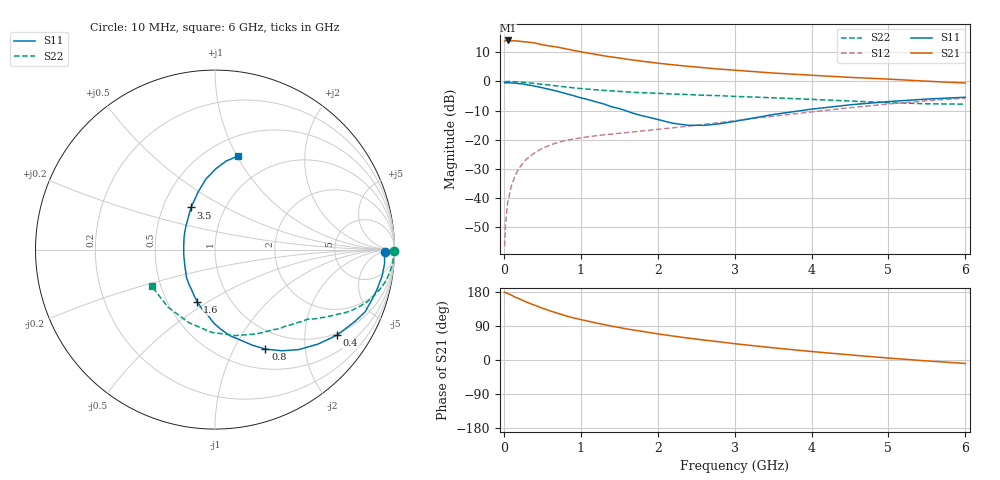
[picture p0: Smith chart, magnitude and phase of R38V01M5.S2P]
! SIEMENS Small Signal Semiconductors
! BFR181
! Si NPN RF Bipolar Junction Transistor in SOT23
! VCE = 8 V  IC = 1.5 mA
! Common Emitter S-Parameters:  May  1996
# GHz  S  MA  R  50
!  f  S11  S21  S12  S22
! GHz  MAG  ANG  MAG  ANG  MAG  ANG  MAG  ANG
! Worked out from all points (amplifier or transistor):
!   36 points, 10 MHz to 6 GHz, reference 50 ohm
!   highest |S21| = 14.0 dB at 50 MHz (marker M1)
!   |S21| within 3 dB of that: start of sweep to 830.6 MHz
!   unconditionally stable (mu >= 1): 1.833 GHz to 3.565 GHz
!   at 250 MHz: K = 0.19, MSG = 20.8 dB, |S12| = -27.9 dB
!   at 1.4 GHz: K = 0.86, MSG = 13.2 dB, |S12| = -18.1 dB
!   at 6 GHz: K = 0.86, MSG = 2.6 dB, |S12| = -5.7 dB
!   S11 on the Smith chart (normalised r, x): 10 MHz: 34, -10; 400 MHz: 0.94, -2.90; 800 MHz: 0.74, -1.35; 1.6 GHz: 0.70, -0.45; 3.5 GHz: 0.69, +0.35; 6 GHz: 0.69, +1.01
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0.01  0.9475 -0.9  4.937 179.0  0.0015 89.8  0.9981 -0.5
0.02  0.9451 -1.8  4.979 177.8  0.0033 91.1  0.9883 -0.9
0.05  0.9481 -4.7  5.032 175.4  0.0084 87.4  0.9956 -2.2
0.1  0.9423 -9.1  4.944 171.1  0.0164 83.0  0.9931 -4.3
0.15  0.9292 -14.0  4.969 165.5  0.0249 81.0  0.9845 -6.6
0.3  0.8775 -27.0  4.743 152.4  0.0472 73.7  0.9524 -12.6
0.4  0.8307 -35.0  4.563 144.8  0.0597 68.8  0.9236 -16.1
0.5  0.778 -42.6  4.239 136.6  0.0711 64.7  0.8931 -19.2
0.6  0.7272 -50.0  4.043 129.8  0.0812 61.2  0.8633 -21.7
0.7  0.6752 -56.6  3.863 123.2  0.0894 58.4  0.8337 -24.0
0.8  0.6215 -63.1  3.63 117.0  0.0968 56.0  0.8049 -25.9
0.9  0.5724 -68.6  3.414 111.3  0.1026 54.2  0.7769 -27.5
1.1  0.4864 -80.2  3.053 102.2  0.1127 51.7  0.7352 -30.4
1.4  0.3686 -96.2  2.617 89.4  0.125 50.1  0.6882 -33.9
1.6  0.3092 -108.4  2.399 81.8  0.1331 49.9  0.6619 -35.8
1.9  0.2401 -127.6  2.136 72.3  0.1458 50.8  0.6317 -39.0
2.2  0.1913 -151.3  1.926 63.2  0.1604 51.9  0.6078 -42.3
2.6  0.1763 171.3  1.717 52.7  0.1842 53.1  0.5788 -47.5
3.5  0.2704 119.6  1.392 32.2  0.2523 52.4  0.524 -63.7
4.5  0.3968 97.3  1.173 13.5  0.3539 46.0  0.4613 -92.4
5.5  0.4982 82.7  1.008 -2.4  0.4655 34.1  0.4138 -129.4
6  0.5354 76.3  0.937 -9.1  0.5171 26.7  0.4072 -149.7
